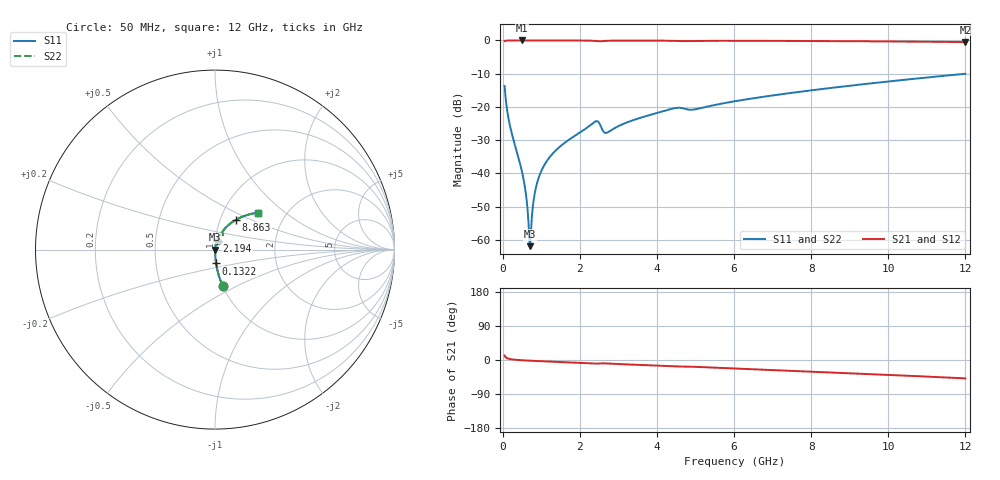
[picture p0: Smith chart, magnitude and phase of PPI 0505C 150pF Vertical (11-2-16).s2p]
# GHz S MA R 50
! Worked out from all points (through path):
!   1601 points, 50 MHz to 12 GHz, reference 50 ohm
!   highest |S21| = -0.01 dB at 505.6 MHz (marker M1); lowest = -0.5 dB at 12 GHz (marker M2)
!   group delay of S21, straight-line fit = 11.3 ps
!   lowest |S11| = -61.9 dB at 707.2 MHz (marker M3), VSWR 1.00, Z = 50.1 - j0.00109 ohm
!   |S11| at or under -10 dB: start of sweep to end of sweep
!   |S22| runs from -61.9 to -10.0 dB; largest |S21 - S12| = 0
!   S11 on the Smith chart (normalised r, x): 50 MHz: 1.00, -0.42; 132.2 MHz: 1.00, -0.15; 2.194 GHz: 1.02, +0.10; 8.863 GHz: 1.19, +0.41; 12 GHz: 1.45, +0.66
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0.05  0.2063 -78.1  0.9782 11.8  0.9782 11.8  0.2063 -78.1
0.1321563  0.07713 -85.6  0.9966 4.1  0.9966 4.1  0.07713 -85.6
0.22925  0.04133 -87.5  0.9986 1.8  0.9986 1.8  0.04133 -87.5
0.5055937  0.01029 -86.8  0.9992 -0.7  0.9992 -0.7  0.01029 -86.8
0.5952188  0.005254 -83.1  0.9992 -1.2  0.9992 -1.2  0.005254 -83.1
0.6699063  0.001801 -65.8  0.9992 -1.6  0.9992 -1.6  0.001801 -65.8
0.70725  0.0008032 -0.8  0.9992 -1.8  0.9992 -1.8  0.0008032 -0.8
0.7445938  0.001771 60.3  0.9991 -2.0  0.9991 -2.0  0.001771 60.3
0.8043438  0.004005 75.4  0.9991 -2.3  0.9991 -2.3  0.004005 75.4
0.8640937  0.006181 79.2  0.999 -2.6  0.999 -2.6  0.006181 79.2
1.058281  0.01266 82.2  0.9989 -3.4  0.9989 -3.4  0.01266 82.2
1.416781  0.02333 82.2  0.9985 -5.0  0.9985 -5.0  0.02333 82.2
2.044156  0.04271 79.0  0.9965 -7.7  0.9965 -7.7  0.04271 79.0
2.193531  0.04898 76.8  0.9946 -8.4  0.9946 -8.4  0.04898 76.8
2.44  0.06106 61.1  0.978 -9.6  0.978 -9.6  0.06106 61.1
2.701406  0.04088 63.5  0.9869 -9.2  0.9869 -9.2  0.04088 63.5
4.038312  0.08223 72.1  0.9923 -15.1  0.9923 -15.1  0.08223 72.1
6.025  0.1218 65.9  0.9884 -22.4  0.9884 -22.4  0.1218 65.9
8.019156  0.178 58.3  0.9802 -30.6  0.9802 -30.6  0.178 58.3
8.863125  0.2038 54.8  0.975 -34.2  0.975 -34.2  0.2038 54.8
10.01331  0.2416 49.9  0.9661 -39.3  0.9661 -39.3  0.2416 49.9
12  0.3152 40.7  0.9441 -48.5  0.9441 -48.5  0.3152 40.7
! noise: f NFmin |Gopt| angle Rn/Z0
0.05  0.0003789  0.8611  0.2643  0.0005844
1.372  0.00399  0.6743  3.433  0.00236
2.701  0.01813  0.8447  6.911  0.02471
4.031  0.01278  0.6979  10.03  0.00821
5.36  0.01759  0.7071  13.35  0.01165
6.682  0.01541  0.6087  16.01  0.007161
8.012  0.01687  0.5806  18.77  0.00714
9.341  0.01885  0.5681  21.51  0.007629
10.67  0.0211  0.5631  24.2  0.008338
12  0.02357  0.5632  26.85  0.009229
